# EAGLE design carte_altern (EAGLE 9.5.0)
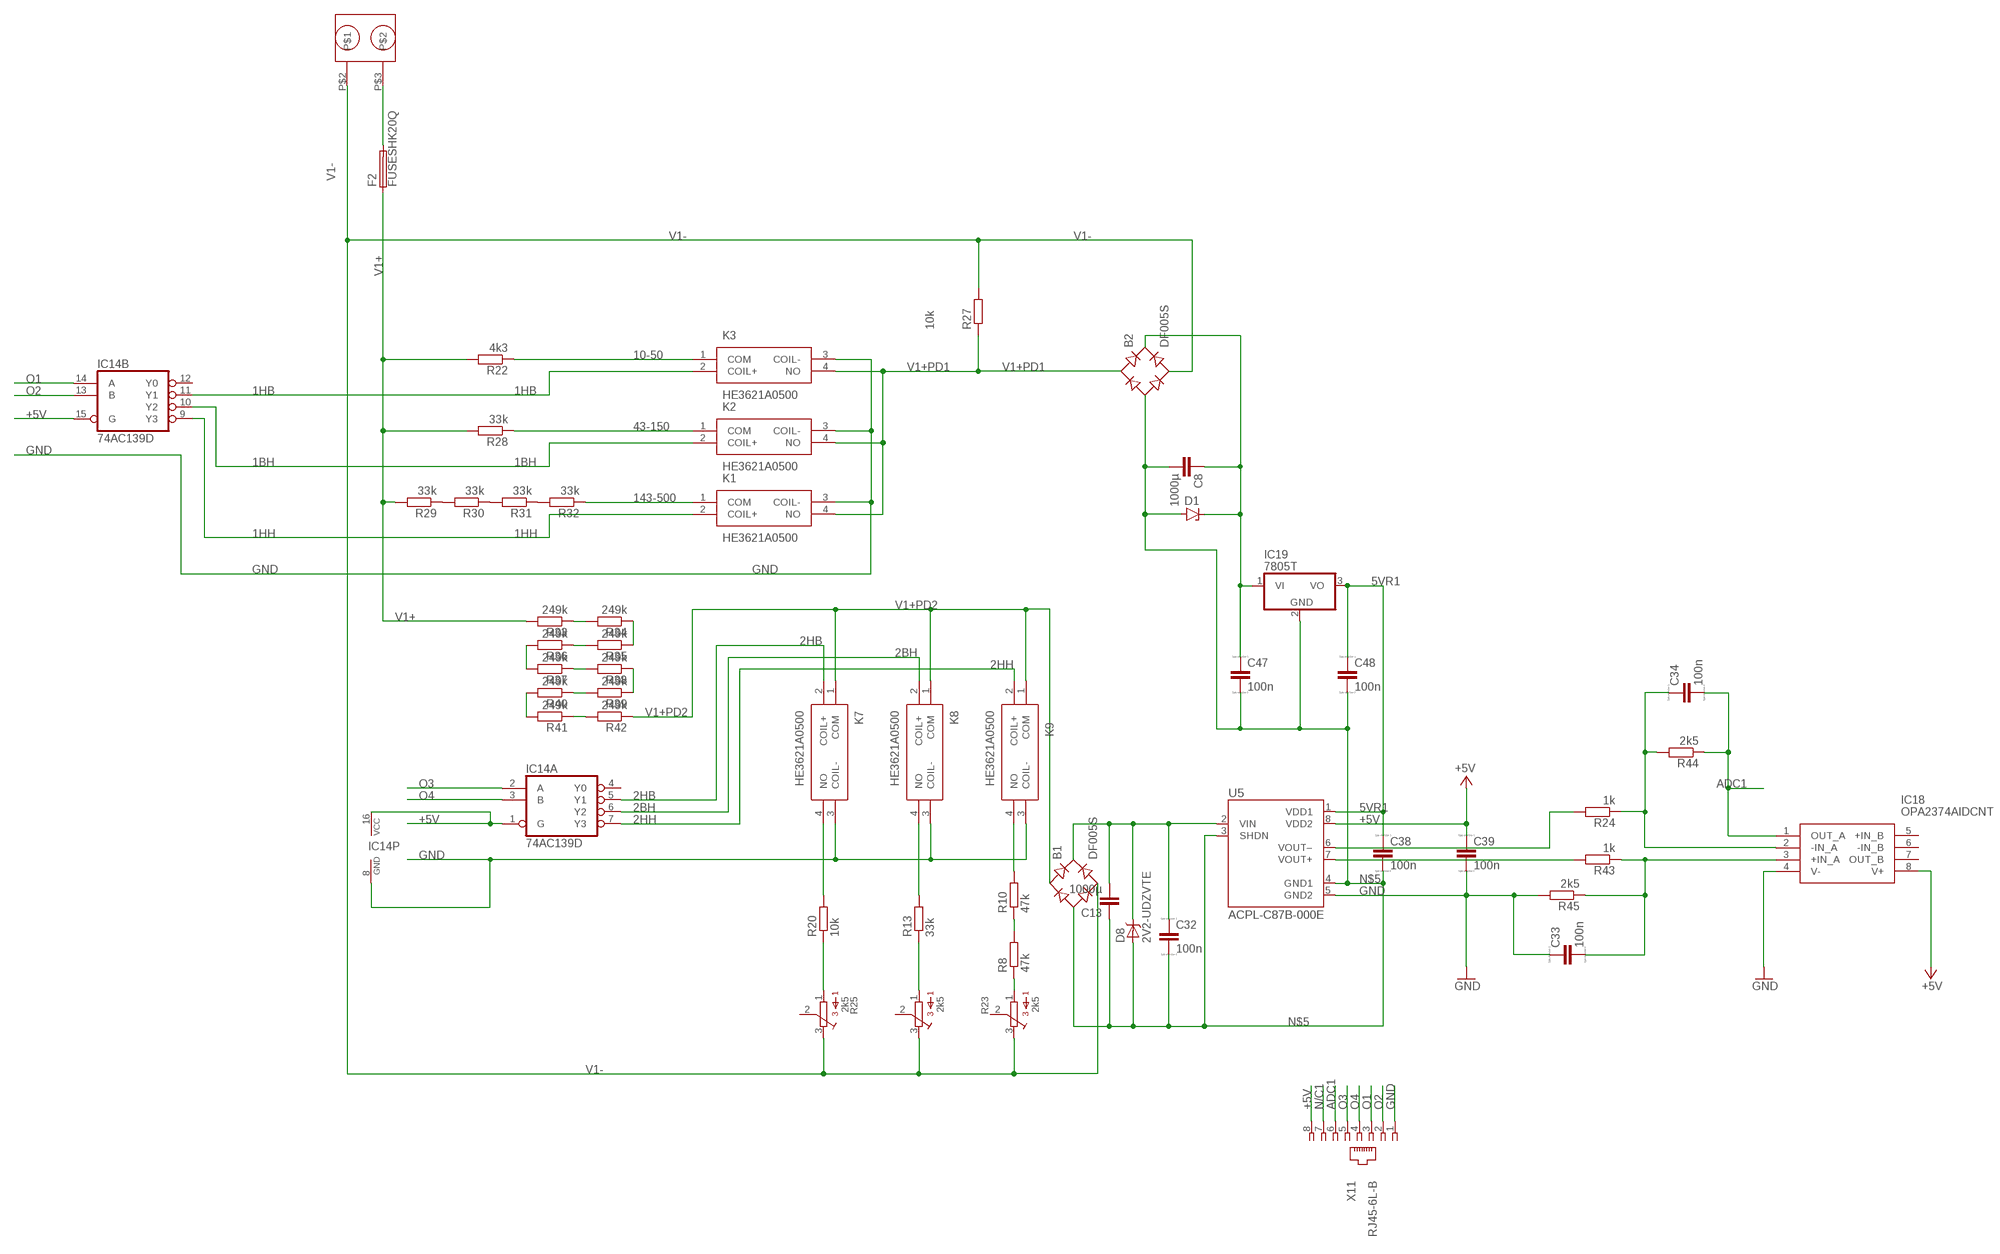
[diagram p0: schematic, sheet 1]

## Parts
B1  DF005S  [DFS]
B2  DF005S  [DFS]
C8  1000µ  C-EU050-075X075  [C050-075X075]
C13  1000µ  C-EU050-075X075  [C050-075X075]
C32  100n  CC2012  [C2012]
C33  100n  CC2012  [C2012]
C34  100n  CC2012  [C2012]
C38  100n  CC2012  [C2012]
C39  100n  CC2012  [C2012]
C47  100n  CC2012  [C2012]
C48  100n  CC2012  [C2012]
D1  ZENER-DIODEDO41Z10  [DO41Z10]
D8  2V2-UDZVTE  BAS70J  [SOD-323]
F2  FUSESHK20Q  [SHK20Q]
IC14  74AC139D  [SO16]
IC18  OPA2374AIDCNT  [SOT65P280X145-8N]
IC19  7805T  [TO220H]
K1  HE3621A0500  [HE3621A0500]
K2  HE3621A0500  [HE3621A0500]
K3  HE3621A0500  [HE3621A0500]
K7  HE3621A0500  [HE3621A0500]
K8  HE3621A0500  [HE3621A0500]
K9  HE3621A0500  [HE3621A0500]
R8  47k  R-EU_M0805  [M0805]
R10  47k  R-EU_M0805  [M0805]
R13  33k  R-EU_M0805  [M0805]
R20  10k  R-EU_M0805  [M0805]
R21  2k5  3362P  [3362P]
R22  4k3  R-EU_M0805  [M0805]
R23  2k5  3362P  [3362P]
R24  1k  R-EU_M0805  [M0805]
R25  2k5  3362P  [3362P]
R27  10k  R-EU_M0805  [M0805]
R28  33k  R-EU_M0805  [M0805]
R29  33k  R-EU_M0805  [M0805]
R30  33k  R-EU_M0805  [M0805]
R31  33k  R-EU_M0805  [M0805]
R32  33k  R-EU_M0805  [M0805]
R33  249k  R-EU_M0805  [M0805]
R34  249k  R-EU_M0805  [M0805]
R35  249k  R-EU_M0805  [M0805]
R36  249k  R-EU_M0805  [M0805]
R37  249k  R-EU_M0805  [M0805]
R38  249k  R-EU_M0805  [M0805]
R39  249k  R-EU_M0805  [M0805]
R40  249k  R-EU_M0805  [M0805]
R41  249k  R-EU_M0805  [M0805]
R42  249k  R-EU_M0805  [M0805]
R43  1k  R-EU_M0805  [M0805]
R44  2k5  R-EU_M0805  [M0805]
R45  2k5  R-EU_M0805  [M0805]
U5  ACPL-C87B-000E  [SOIC127P1150X360-8N]
U$20  BORNIER-508  [BORNIER-508_FOOTPRINT]
X11  RJ45-6L-B  [RJ45-NO-SHIELD]

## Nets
1BH: IC14.10(B:Y2) K2.2(COIL+)
1HB: IC14.11(B:Y1) K3.2(COIL+)
1HH: IC14.9(B:Y3) K1.2(COIL+)
2BH: IC14.6(A:Y2) K8.2(COIL+)
2HB: IC14.5(A:Y1) K7.2(COIL+)
2HH: IC14.7(A:Y3) K9.2(COIL+)
5VR1: C38.1 C48.1 IC19.3(VO) U5.1(VDD1)
10-50: K3.1(COM) R22.1
43-150: K2.1(COM) R28.1
143-500: K1.1(COM) R32.1
+5V [power]: C39.1 IC14.1(A:G) IC14.15(B:G) IC14.16(P:VCC) IC18.8(V+) U5.8(VDD2) X11.8
ADC1: C34.2 IC18.1(OUT_A) R44.1 X11.6
GND: C33.1 C39.2 IC14.8(P:GND) IC18.4(V-) K1.3(COIL-) K2.3(COIL-) K3.3(COIL-) K7.3(COIL-) K8.3(COIL-) K9.3(COIL-) R45.2 U5.5(GND2) X11.1
N$1: B1.+ C13.2 C32.1 D8.C U5.2(VIN)
N$2: F2.2A U$20.P$3
N$5: B1.- B2.- C8.2 C13.1 C32.2 C38.2 C47.2 C48.2 D1.A D8.A IC19.2(GND) U5.3(SHDN) U5.4(GND1)
N$13: K7.4(NO) R20.2
N$14: R8.2 R10.1
N$15: R8.1 R23.1
N$18: K9.4(NO) R10.2
N$58: R20.1 R25.1
N$69: C33.2 IC18.3(+IN_A) R43.1 R45.1
N$70: R41.1 R42.2
N$71: R39.2 R40.1
N$72: R37.1 R38.2
N$73: R35.2 R36.1
N$74: R33.1 R34.2
N$75: R34.1 R35.1
N$76: R36.2 R37.2
N$77: R38.1 R39.1
N$78: R40.2 R41.2
N$82: R43.2 U5.7(VOUT+)
N$83: R24.2 U5.6(VOUT–)
N$84: C34.1 IC18.2(-IN_A) R24.1 R44.2
N$87: B2.+ C8.1 C47.1 D1.C IC19.1(VI)
N$100: R29.1 R30.2
N$101: R30.1 R31.2
N$102: R31.1 R32.2
N$106: R13.1 R21.1
N$107: K8.4(NO) R13.2
N/C1: X11.7
O1: IC14.14(B:A) X11.3
O2: IC14.13(B:B) X11.2
O3: IC14.2(A:A) X11.5
O4: IC14.3(A:B) X11.4
V1+: F2.1A R22.2 R28.2 R29.2 R33.2
V1+PD1: B2.AC1 K1.4(NO) K2.4(NO) K3.4(NO) R27.1
V1+PD2: B1.AC1 K7.1(COM) K8.1(COM) K9.1(COM) R42.1
V1-: B1.AC2 B2.AC2 R21.3 R23.3 R25.3 R27.2 U$20.P$2
Unconnected: IC14.4(A:Y0) IC14.12(B:Y0) IC18.5(+IN_B) IC18.6(-IN_B) IC18.7(OUT_B) R21.2 R23.2 R25.2

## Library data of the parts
B1 B2 = rectifier:DF*S: Surface Mount Glass Passivated Bridge Rectifiers Source: Source: Comchip Bridge Rectifiers DF005S-G thru DF10S-G.pdf
C8 C13 = rcl:C-EU: CAPACITOR, European symbol; SPICEPREFIX: C
C32-C34 C38 C39 C47 C48 = eagle-ltspice:C: CAPACITOR, European symbol; SPICEMODEL: NONE; SPICEPREFIX: C
D1 = diode:ZENER-DIODE: Z-Diode
D8 = ELL-i-DiscreteSemi:BAS70: Silicon Schottky Diodes
F2 = fuse:FUSE: Fuse; OC_FARNELL: unknown; OC_NEWARK: unknown
IC14 = 74xx-eu:74*139: Dual 2-line to 4-line DECODER/DEMULTIPLEXER; SPICEPREFIX: I
IC18 = OPA2374AIDCNT:OPA2374AIDCNT: Texas Instruments OPA2374AIDCNT, Dual Op Amp, 6.5MHz CMOS, Rail to Rail, 3 V, 5 V, 8-Pin SOT-23 Source: Datasheet; DESCRIPTION: Texas Instruments OPA2374AIDCNT, Dual Op Amp, 6.5MHz CMOS, Rail to Rail, 3 V, 5 V, 8-Pin SOT-23; HEIGHT: mm; MANUFACTURER_NAME: Texas Instruments; MANUFACTURER_PART_NUMBER: OPA2374AIDCNT; MOUSER_PART_NUMBER: 595-OPA2374AIDCNT; MOUSER_PRICE-STOCK: https://www.mouser.com/Search/Refine.aspx?Keyword=595-OPA2374AIDCNT
IC19 = linear:78*: Positive VOLTAGE REGULATOR Source: http://cache.national.com/ds/LM/LM78L05.pdf http://www.fairchildsemi.com/ds/LM/LM7805.pdf
K1-K3 K7-K9 = HE3621A0500:HE3621A0500: Reed Relays REED RELAY Source: Datasheet; DESCRIPTION: Reed Relays REED RELAY; HEIGHT: 7mm; MANUFACTURER_NAME: Hamlin / Littelfuse; MANUFACTURER_PART_NUMBER: HE3621A0500; MOUSER_PART_NUMBER: 934-HE3621A0500; MOUSER_PRICE-STOCK: https://www.mouser.com/Search/Refine.aspx?Keyword=934-HE3621A0500
R8 R10 R13 R20 R22 R24 R27-R45 = rcl:R-EU_: RESISTOR, European symbol; SPICEPREFIX: R
R21 R23 R25 = bourns:3362: 3362 Series 1/4" Square Trimmer
U5 = ACPL-C87B-000E:ACPL-C87B-000E: Precision Optically Isolated Voltage Sensor; AVAILABILITY: Unavailable; DESCRIPTION: Isolation Amplifier, Optically, 1, 9.9 mV, 5 kV, 3V to 5.5V, SOIC, 8; MF: Broadcom Limited; MP: ACPL-C87B-000E; PACKAGE: SO-8 Broadcom; PRICE: None
U$20 = bornier-508:BORNIER-508
X11 = con-tycoelectronics:RJ45: CORCOM Modular RJ Jacks No Shield Source: www.tycoelectronics.com .. ENG_DS_1654001_1099_RJ_L_0507.pdf; MPN: RJ45-6L-B; OC_FARNELL: unknown; OC_NEWARK: 16R6090

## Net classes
0 default: width 0.152 mm, drill 0.61 mm, clearance 0.152 mm
1 power: width 0.152 mm, drill 0.61 mm, clearance 0.152 mm
2 VIN: width 0.61 mm, drill 0.61 mm, clearance 0.254 mm

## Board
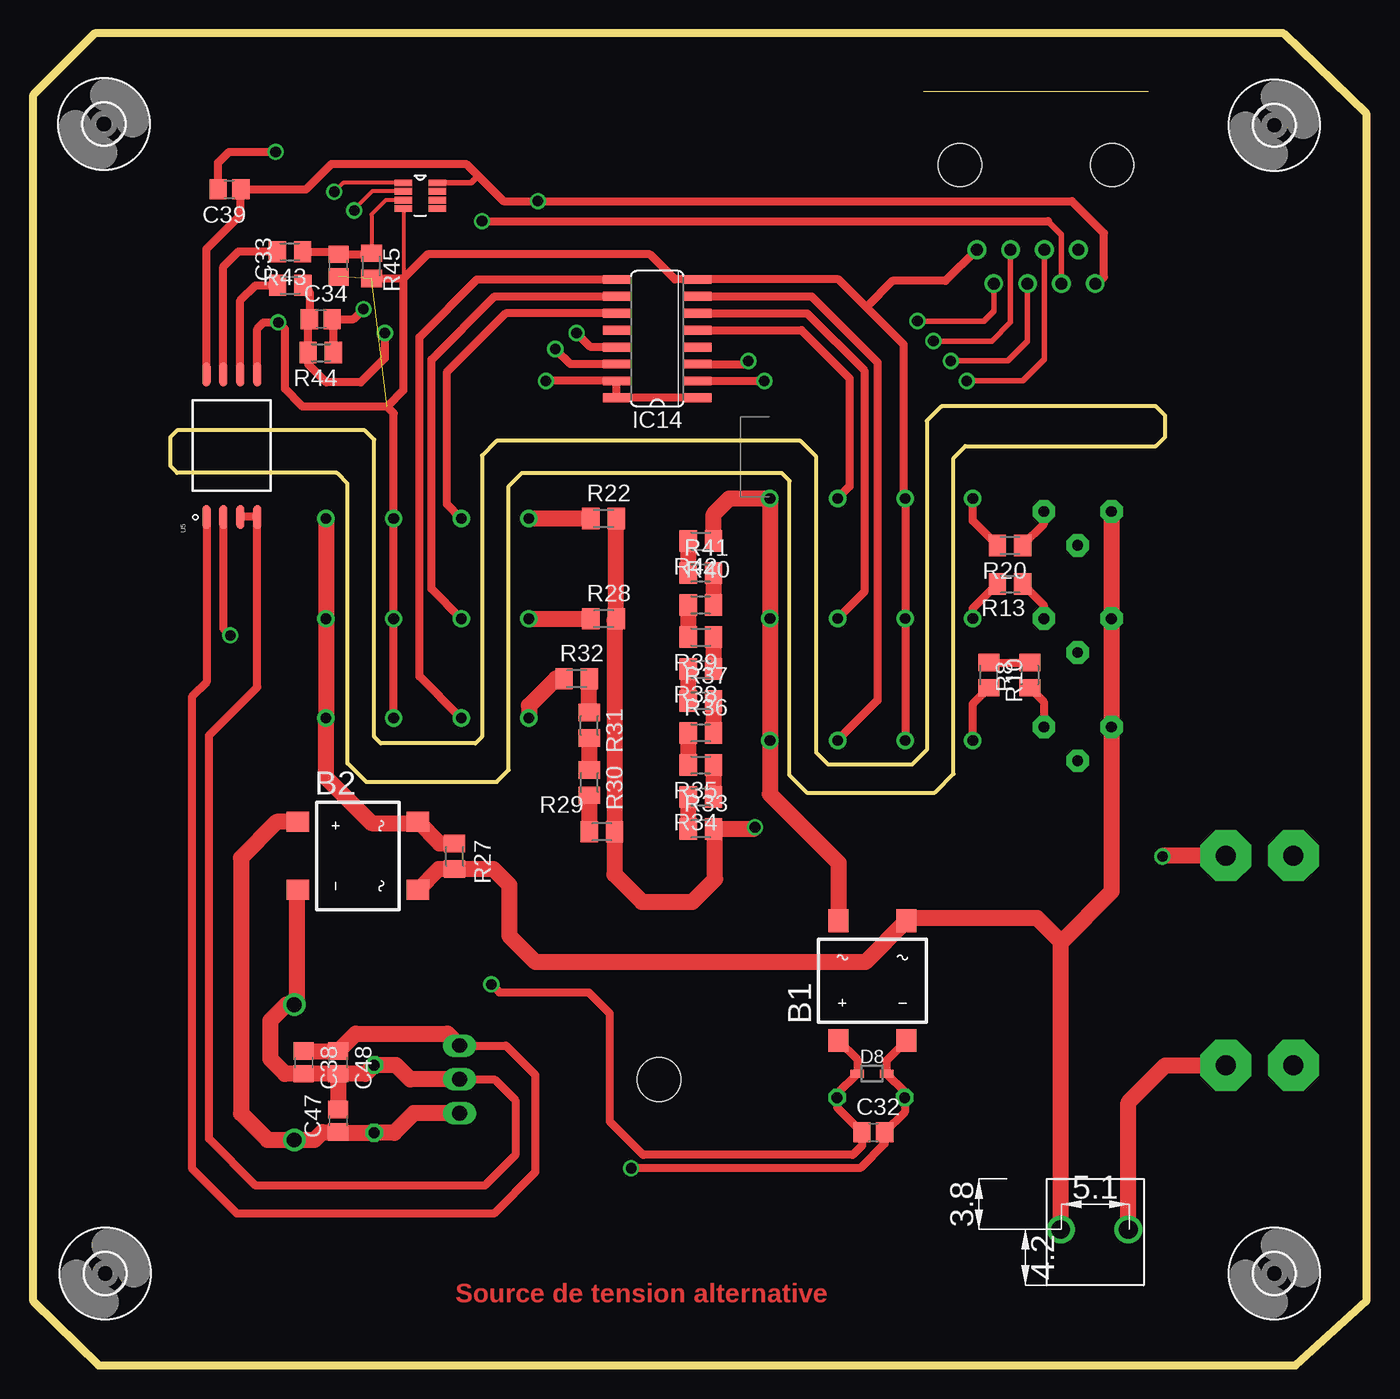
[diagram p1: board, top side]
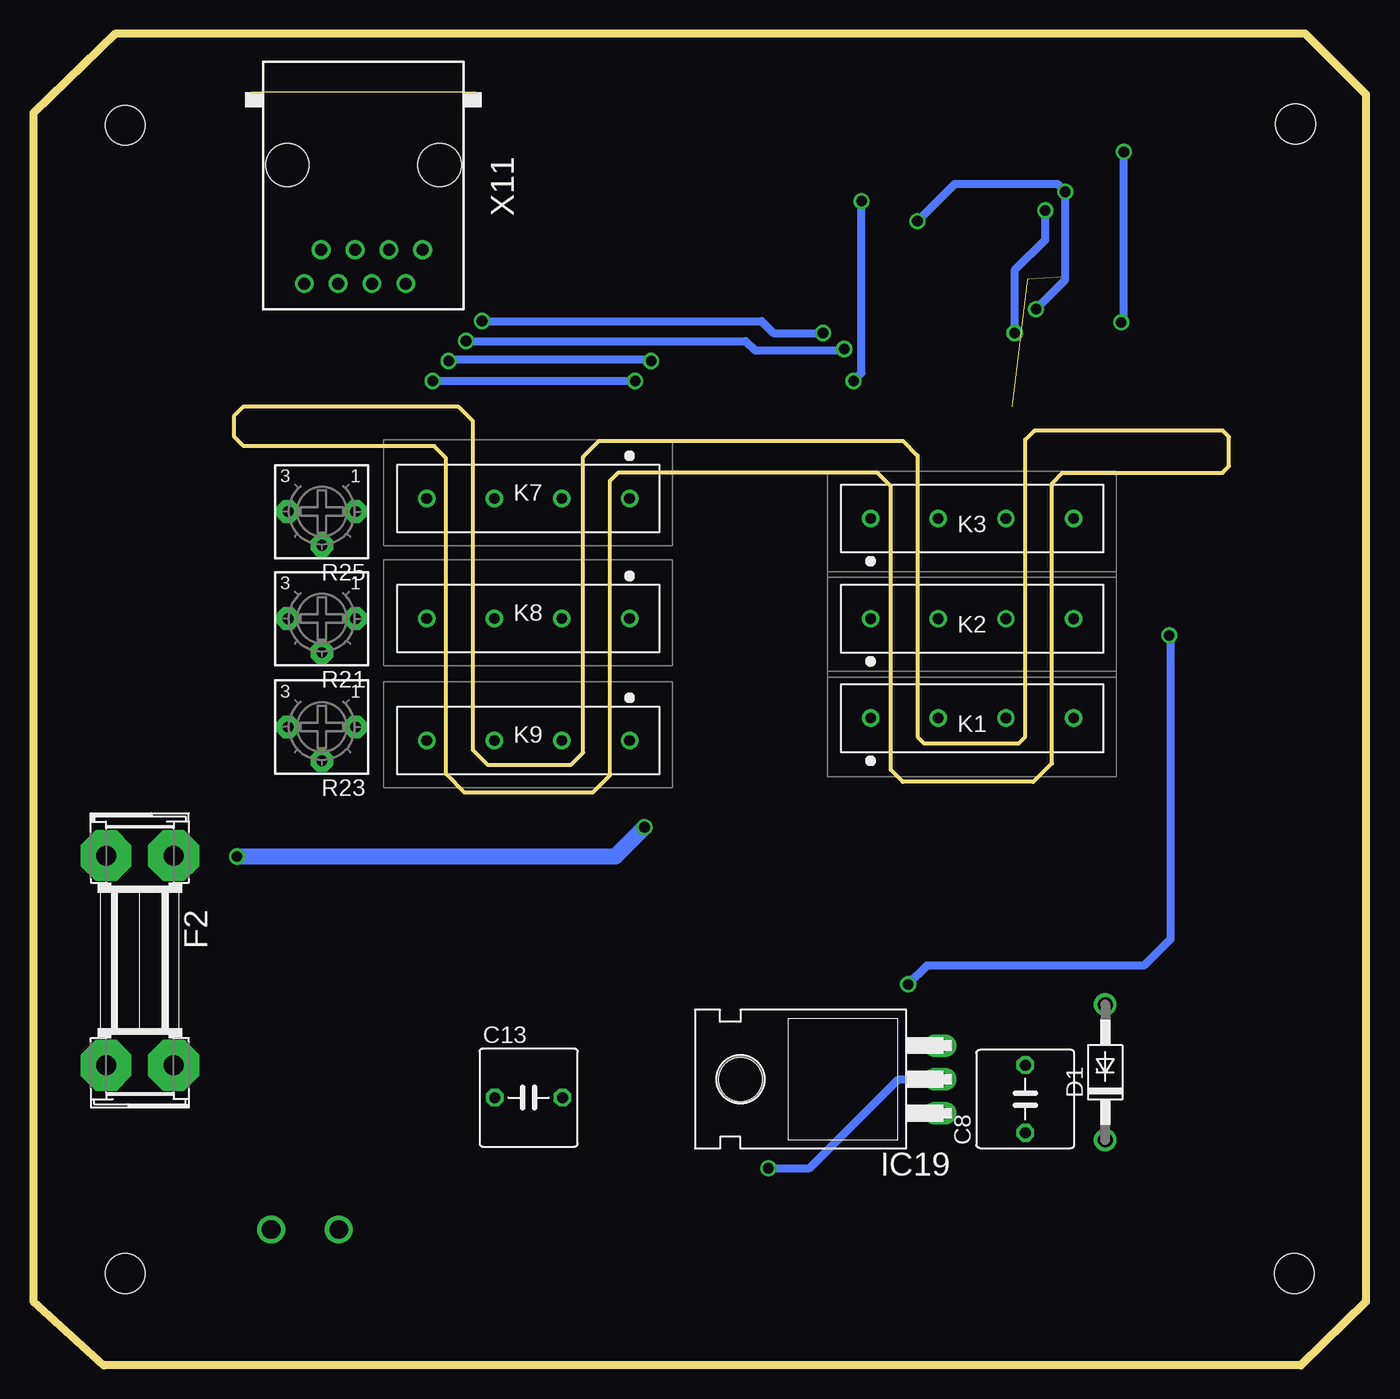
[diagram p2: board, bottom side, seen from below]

Size 100.1 x 100 mm. Coordinates in mm from the lower left corner, seen from the top.
Outline: 25.6,47.2 25.6,69.5 24.9,70.2 10.8,70.2 10.3,69.7 10.3,67.5 10.8,67 22.8,67 23.6,66.2 23.6,45.2 25,43.8 34.8,43.8 35.7,44.7 35.7,66 36.7,67 56.2,67 56.8,66.4 56.8,44.3 58.1,43 67.7,43 69.1,44.4 69.1,68.1 70,69 84.3,69 85,69.7 85,71.3 84.3,72 68.2,72 67.1,70.9 67.1,46.2 66,45.1 59.7,45.1 58.8,46 58.8,68.2 57.6,69.4 34.8,69.4 33.7,68.3 33.7,47.2 33.2,46.7 26.1,46.7 25.6,47.2
Outline: 100.1,4.8 94.8,0 4.9,0 0,4.8 0,95.4 4.6,100 93.9,100 100.1,94 100.1,4.8
Copper layers (1*16): Top 0.035mm / dielectric 1.5mm / Bottom 0.035mm
Design rules "ArduinoETH *": minimum track width 0.2mm, minimum drill 0.8mm, track to track 0.3mm, track to pad 0.3mm, pad to pad 0.2mm, via to via 0.2mm, smd to smd 0.3mm, copper to edge 25mil, drill to drill 10mil, minimum pad ring 10mil, minimum via ring 8mil, stop-mask expansion 1mil, vias tented up to drill 30mil, thermal gap 10mil

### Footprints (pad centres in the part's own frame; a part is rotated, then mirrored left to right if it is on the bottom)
DFS = smd 1.5 x 1.7: + -2.55,-4.5; - 2.55,-4.5; AC1 -2.55,4.5; AC2 2.55,4.5
C050-075X075 = drill 0.813 octagon: 1 -2.54,0; 2 2.54,0
C2012 = smd 1.3 x 1.5: 1 -0.85,0; 2 0.85,0
DO41Z10 = drill 1.118: A 5.08,0; C -5.08,0
SOD-323 = smd 1 x 0.6: A 1.1,0; C -1.1,0
SHK20Q = drill 1.5 pad 3.81 octagon: 1A -7.874,2.54; 1B -7.874,-2.54; 2A 7.874,2.54; 2B 7.874,-2.54
SO16 = smd 0.66 x 2.032: 1 -4.445,-3.073; 2 -3.175,-3.073; 3 -1.905,-3.073; 4 -0.635,-3.073; 5 0.635,-3.073; 6 1.905,-3.073; 7 3.175,-3.073; 8 4.445,-3.073; 9 4.445,3.073; 10 3.175,3.073; 11 1.905,3.073; 12 0.635,3.073; 13 -0.635,3.073; 14 -1.905,3.073; 15 -3.175,3.073; 16 -4.445,3.073
SOT65P280X145-8N = smd 1.321 x 0.508: 1 -1.27,0.965; 2 -1.27,0.33; 3 -1.27,-0.33; 4 -1.27,-0.965; 5 1.27,-0.965; 6 1.27,-0.33; 7 1.27,0.33; 8 1.27,0.965
TO220H = drill 1.118 long: 1 -2.54,-10.16; 2 0,-10.16; 3 2.54,-10.16 | hole 3.302: 0,4.826
HE3621A0500 = drill 0.8 pad 1.3: 1 0,0; 2 5.08,0; 3 10.16,0; 4 15.24,0
M0805 = smd 1.3 x 1.6: 1 -0.95,0; 2 0.95,0
3362P = drill 0.813 pad 1.676 octagon: 1 -2.54,0; 2 0,2.54; 3 2.54,0
SOIC127P1150X360-8N = smd 1.8 x 0.6: 1 -5.35,1.905; 2 -5.35,0.635; 3 -5.35,-0.635; 4 -5.35,-1.905; 5 5.35,-1.905; 6 5.35,-0.635; 7 5.35,0.635; 8 5.35,1.905
3,0 = hole 3: 0,0
BORNIER-508_FOOTPRINT = drill 1.4: P$2 -0.04,0; P$3 5.04,0
RJ45-NO-SHIELD = drill 0.9 pad 1.4: 1 -4.445,6.35; 2 -3.175,8.89; 3 -1.905,6.35; 4 -0.635,8.89; 5 0.635,6.35; 6 1.905,8.89; 7 3.175,6.35; 8 4.445,8.89 | hole 3.251: -5.715,0; 5.715,0

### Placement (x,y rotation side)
B1  63.02,28.88 0 top
B2  24.38,38.24 270 top
C8  25.6,20 90 bottom
C13  62.9,20.1 0 bottom
C32  63.08,17.5 0 top
C33  22.92,82.57 90 top
C34  21.6,78.54 0 top
C38  20.31,22.74 270 top
C39  14.73,88.28 180 top
C47  22.91,18.36 90 top
C48  22.9,22.74 270 top
D1  19.6,22 90 bottom
D8  62.98,21.9 0 top
F2  92.1,30.4 270 bottom
IC14  46.86,77.08 90 top
IC18  29.06,87.81 0 top
IC19  42.17,21.47 90 bottom
K1  37.22,48.59 0 bottom
K2  37.22,56.05 0 bottom
K3  37.22,63.57 0 bottom
K7  55.32,65.08 180 bottom
K8  55.32,56.06 180 bottom
K9  55.32,46.91 180 bottom
R8  74.84,51.81 90 top
R10  71.76,51.81 270 top
R13  73.35,58.66 180 top
R20  73.35,61.56 180 top
R21  78.43,56.06 180 bottom
R22  42.83,63.57 0 top
R23  78.43,47.92 180 bottom
R24  19.3,81.09 180 top
R25  78.43,64.1 180 bottom
R27  31.64,38.22 270 top
R28  42.83,56.05 0 top
R29  42.7,40.06 0 top
R30  41.75,43.75 270 top
R31  41.75,48.05 270 top
R32  40.8,51.55 0 top
R33  50.13,40.27 0 top
R34  50.13,42.67 180 top
R35  50.13,45.07 180 top
R36  50.13,47.47 0 top
R37  50.13,49.87 0 top
R38  50.13,52.27 180 top
R39  50.13,54.67 180 top
R40  50.13,57.07 0 top
R41  50.13,59.47 0 top
R42  50.13,61.87 180 top
R43  19.28,83.6 180 top
R44  21.6,76.03 180 top
R45  25.4,82.54 270 top
U5  14.91,69.04 90 top
U$2  [3,0]  5.4,6.9 180 top
U$3  [3,0]  5.3,93.2 180 top
U$6  [3,0]  93.2,93.1 180 top
U$7  [3,0]  93.2,6.9 180 top
U$20  77.2,10.2 0 top
X11  75.3,90.1 180 bottom

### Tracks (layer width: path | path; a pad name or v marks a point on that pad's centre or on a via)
1BH
  Top 0.6: K2.2 29.9,58.29 29.9,75.5 34.65,80.25 IC14.10
1HB
  Top 0.6: IC14.11 35.48,78.98 31.04,74.54 31.04,64.67 K3.2
1HH
  Top 0.6: K1.2 29,51.73 29,77.2 33.32,81.52 IC14.9
2BH
  Top 0.6: IC14.6 58.12,78.98 62.4,74.7 62.4,58.06 K8.2
2HB
  Top 0.6: IC14.5 57.69,77.71 61.3,74.1 61.3,65.98 K7.2
2HH
  Top 0.6: IC14.7 58.45,80.25 63.4,75.3 63.4,49.91 K9.2
5VR1
  Top 0.6: U5.1 13.01,51.29 11.9,50.19 11.9,14.8 15.3,11.4 34.6,11.4 37.7,14.5 37.7,21.8 35.49,24.01 IC19.3
  Top 1.2: C38.1 C48.1 24.22,24.91 31.11,24.91 IC19.3
10-50
  Top 1.2: R22.1 K3.1
43-150
  Top 1.2: K2.1 R28.1
143-500
  Top 1.2: R32.1 39.25,51.55 37.22,49.52 K1.1
+5V  (via drill 0.8)
  Top 0.4: IC18.8 32.87,88.77 33.4,89.3
  Top 0.6: v38.5,73.9 IC14.15 IC14.16 IC14.1 | U5.8 13.01,83.81 15.58,86.38 C39.1 20.47,88.28 22.4,90.2 32.5,90.2 33.4,89.3 35.3,87.4 v37.9,87.4 78,87.4 80.4,85 80.4,81.7 79.91,81.21 X11.8
  Bottom 0.6: v38.5,73.9 37.9,74.5 v37.9,87.4
ADC1  (via drill 0.8)
  Top 0.3: IC18.1 23.27,88.77 v22.6,88.1
  Top 0.4: X11.6 77.2,84.9 76.2,85.9
  Top 0.6: R44.1 22.55,78.44 C34.2 24.04,78.54 v24.8,79.3 | v33.7,85.9 76.2,85.9
  Bottom 0.6: v24.8,79.3 22.6,81.5 v22.6,88.1 23.2,88.7 30.9,88.7 v33.7,85.9
GND  (via drill 0.8)  (2 unrouted)
  Top 0.3: IC18.4 27.79,81.59
  Top 0.6: K9.3 K8.3 K7.3 65.38,65.18 65.38,76.62 62.55,79.45 | K1.3 K2.3 K3.3 27.06,71.46 26.56,71.96 | 62.55,79.45 60.48,81.52 IC14.8 48.18,81.52 46.3,83.4 29.6,83.4 27.79,81.59 | 27.79,81.59 R45.2 | 27.79,81.59 27.79,73.19 26.6,72 20.2,72 18.9,73.3 18.9,77.8 v18.4,78.3 17.3,78.3 16.82,77.82 U5.5 | X11.1 68.51,81.41 64.51,81.41 62.55,79.45 | C39.2 13.88,90.28 14.7,91.1 v18.2,91.1
  Bottom 0.6: v18.4,78.3 18.2,78.5 v18.2,91.1
N$1  (via drill 0.8)
  Top 0.6: B1.+ 61.88,22.97 D8.C 60.36,20.38 C13.2 60.36,19.37 C32.1 62.23,16.5 61.54,15.8 45.8,15.8 43.3,18.3 43.3,26.4 41.7,28 35,28 v34.4,28.6 34.3,28.6 | U5.2 14.28,55.32 v14.8,54.8
  Bottom 0.6: v14.8,54.8 14.7,54.7 14.7,32 16.7,30 33,30 v34.4,28.6
N$2
  Top 1.2: U$20.P$3 82.24,19.74 85.03,22.53 F2.2A
N$5  (via drill 0.8)
  Top 0.6: 22.9,19.22 C47.2 | 19,27.08 D1.A 19.78,27.26 | B1.- 64.08,22.88 D8.A 65.44,20.54 C13.1 65.44,19 C32.2 63.93,16.63 62.1,14.8 v44.9,14.8 | U5.3 U5.4 16.82,50.92 13.2,47.3 13.2,17 16.7,13.5 33.9,13.5 36.2,15.8 36.2,19.9 34.63,21.47 IC19.2
  Top 1.2: C48.2 24.95,21.89 C8.2 27.24,22.54 28.31,21.47 IC19.2 | C48.2 C38.2 18.91,21.89 17.8,23 17.8,25.88 19,27.08 | C48.2 22.9,19.22 | B2.- 19.78,35.59 19.78,27.26
  Bottom 0.6: v44.9,14.8 41.8,14.8 35.13,21.47 IC19.2
N$13
  Top 0.6: R20.2 70.56,63.4 K7.4
N$14
  Top 0.6: R10.1 R8.2
N$15
  Top 0.6: R8.1 75.89,49.81 R23.1
N$18
  Top 0.6: K9.4 70.56,49.66 R10.2
N$58
  Top 0.6: R25.1 75.89,63.15 R20.1
N$69
  Top 0.3: IC18.3 26.47,87.47 25.4,86.4 R45.1
  Top 0.6: R43.1 22.73,83.6 C33.2 25.33,83.42 R45.1
N$70
  Top 1.2: R42.2 R41.1
N$71
  Top 1.2: R40.1 R39.2
N$72
  Top 1.2: R38.2 R37.1
N$73
  Top 1.2: R36.1 R35.2
N$74
  Top 1.2: R34.2 R33.1
N$75
  Top 1.2: R35.1 R34.1
N$76
  Top 1.2: R37.2 R36.2
N$77
  Top 1.2: R39.1 R38.1
N$78
  Top 1.2: R41.2 R40.2
N$82
  Top 0.6: R43.2 18.31,83.62 15.42,83.62 14.28,82.48 U5.7
N$83
  Top 0.6: U5.6 15.55,79.95 16.68,81.09 R24.2
N$84  (via drill 0.8)
  Top 0.3: IC18.2 25.43,88.14 24.1,86.8 v24.1,86.7
  Top 0.6: R24.1 20.75,80.59 C34.1 20.65,78.44 R44.2 20.65,75.15 22,73.8 24.6,73.8 26.4,75.6 v26.4,77.5 26.4,77.57
  Bottom 0.6: v26.4,77.5 26.4,82.2 24.1,84.5 v24.1,86.7
N$87
  Top 0.6: C47.1 22.96,17.46
  Top 1.2: 22.96,17.46 C8.1 27.1,17.46 28.57,18.93 IC19.1 | C47.1 21.71,17.51 21.12,16.92 D1.C 17.6,16.92 15.6,18.92 15.6,38.1 18.29,40.79 B2.+
N$100
  Top 0.6: R29.1
  Top 1.2: R29.1 R30.2
N$101
  Top 0.6: R31.2
  Top 1.2: R30.1 R31.2
N$102
  Top 0.6: R32.2
  Top 1.2: R31.1 R32.2
N$106
  Top 0.6: R13.1 75.89,57.06 R21.1
N$107
  Top 0.6: R13.2 70.56,56.82 K8.4
O1  (via drill 0.8)
  Top 0.4: v67.6,76.9 72,76.9 73.39,78.3 X11.3
  Top 0.6: IC14.14 40.33,75.17 v39.2,76.3
  Bottom 0.6: v67.6,76.9 46.6,76.9 45.9,76.2 39.3,76.2 v39.2,76.3
O2  (via drill 0.8)
  Top 0.4: v66.4,78.4 71.4,78.4 72.12,79.12 X11.2
  Top 0.6: IC14.13 41.86,76.44 v40.8,77.5
  Bottom 0.6: v66.4,78.4 45.4,78.4 44.5,77.5 v40.8,77.5
O3  (via drill 0.8)
  Top 0.4: X11.5 75.93,75.53 74.3,73.9 v70.1,73.9
  Top 0.6: v54.9,73.9 IC14.2
  Bottom 0.6: v54.9,73.9 v70.1,73.9
O4  (via drill 0.8)
  Top 0.4: X11.4 74.66,76.87 73.2,75.4 v68.9,75.4
  Top 0.6: IC14.3 53.47,75.17 v53.7,75.4
  Bottom 0.6: v53.7,75.4 53.8,75.5 68.8,75.5 v68.9,75.4
V1+  (via drill 0.8)
  Top 0.6: 51.2,40.16 R33.2 | 54.07,40.27 v54.2,40.4
  Top 1.2: R22.2 R28.2 43.65,55.92 R29.2 43.65,36.85 45.7,34.8 49.5,34.8 51.2,36.5 51.2,40.16 | R33.2 54.07,40.27 | F2.1A 84.87,38.27 v84.8,38.2
  Bottom 1.2: v84.8,38.2 56.4,38.2 v54.2,40.4
V1+PD1
  Top 0.6: K1.4 22.08,48.49 | 31.59,39.12 R27.1
  Top 1.2: K3.4 K2.4 K1.4 21.98,44.12 25.4,40.7 28.79,40.7 B2.AC1 30.5,39.17 R27.1
V1+PD2
  Top 1.2: B1.AC1 60.47,37.73 55.32,42.88 K9.1 K8.1 K7.1 52.28,65.08 51.08,63.88 R42.1
V1-
  Top 1.2: R25.3 R21.3 R23.3 80.97,35.56 77.23,31.82 77.16,31.82 | B2.AC2 30.46,37.27 R27.2 34.53,37.27 35.73,36.07 35.73,32.27 37.72,30.28 62.48,30.28 B1.AC2 65.77,33.58 75.4,33.58 77.16,31.82 | U$20.P$2 77.16,31.82

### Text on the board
Top: Source de tension alternative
